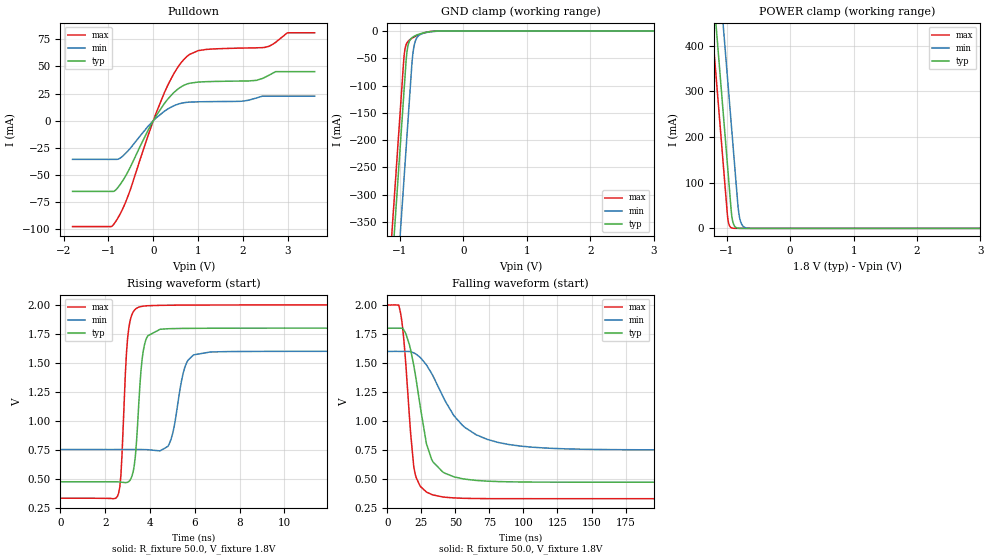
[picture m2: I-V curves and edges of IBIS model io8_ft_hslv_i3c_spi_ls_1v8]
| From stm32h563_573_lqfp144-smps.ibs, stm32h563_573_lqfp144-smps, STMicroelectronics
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[Model]   io8_ft_hslv_i3c_spi_ls_1v8
Model_type I/O_open_drain
Polarity   Non-Inverting
Enable   Active-Low
| CAP_THRESHOLD on pad IOFT is "UDTCAPC" :
| Rising=20.0% of vddiom   Falling=80.0% of vddiom
| C_comp min and max val. don't necessarily correlate with the min and max pvt
| but are the smallest and greatest pad capacitance found.
| var   typ   min   max
C_comp   3.74765pF  3.68522pF  3.87712pF
|C_comp_pulldown   3.74765pF  3.68522pF  3.87712pF
Vinl = 800.0mV
Vinh = 1.0V
Vmeas = 900.0mV   | Reference voltage for timing measurements
Cref  = 50.0pF   | Timing specification test load capacitance value
Rref  = 1.0MOhm   | Timing specification test load resistance value
Vref  = 990.0mV   | Timing specification test load voltage
[Model Spec]
| TIME_THRESHOLD on pin ZII2CV11 is "CMOS" :
| Rising=40.0% of vdd   Falling=60.0% of vdd
Vinl 703.80000mV 631.80000mV 784.80000mV
Vinh 1.06220V 937.20000mV 1.16620V
| variable   typ   min   max
[Temperature Range] 25.0 125.0 -40.0
| variable   typ   min   max
[Voltage Range] 1.8V 1.6V 2.0V
| variable   typ   min   max
[POWER Clamp Reference] 1.8V 1.6V 2.0V
| variable   typ   min   max
[GND Clamp Reference] 0V 0V 0V
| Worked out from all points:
|   slope of the pulldown table from 0 to 0.27 V, typ, clamps not added: 15.8 ohm
|   GND clamp passes 1 mA (typ) near -0.52 V on its own axis
|   POWER clamp passes 1 mA (typ) near -0.84 V on its own axis
|   rising waveform, R_fixture 50.0, V_fixture 1.8V: 20-80 % time 286ps typ, 460ps min, 243ps max; typ from 0.474 V to 1.8 V
|   falling waveform, R_fixture 50.0, V_fixture 1.8V: 20-80 % time 12.1ns typ, 28.6ns min, 6.57ns max; typ from 1.8 V to 0.474 V
[POWER Clamp]
-1.8V     1.518A     1.709A     1.407A
-1.23V    548.8mA    740.2mA    437.5mA
-1.16V    429.8mA    621.2mA    318.5mA
-1.05V    242.8mA    434.2mA    131.5mA
-980mV    123.8mA    315.2mA    17.95mA
-930mV    38.81mA    230.2mA    1.49mA
-910mV    17.82mA    196.2mA    550.8uA
-890mV    8.18mA     162.2mA    203.5uA
-810mV    363.5uA    33.6mA     3.797uA
-770mV    76.62uA    10.47mA    518.8nA
-710mV    7.416uA    1.822mA    26.34nA
3.6V      0A         0A         0A
[GND Clamp]
-1.8V     -1.579A    -1.74A     -1.515A
-1.24V    -627.3mA   -788.3mA   -562.7mA
-1.05V    -304.3mA   -465.3mA   -239.7mA
-940mV    -117.3mA   -278.3mA   -52.69mA
-930mV    -100.3mA   -261.3mA   -40.52mA
-900mV    -50.11mA   -210.3mA   -24.23mA
-880mV    -30.95mA   -176.3mA   -20.02mA
-810mV    -12.18mA   -57.97mA   -13.23mA
-780mV    -9.807mA   -29.1mA    -11.19mA
-690mV    -5.41mA    -7.142mA   -6.184mA
-420mV    -170.4uA   -446.1uA   -81.94uA
3.6V      5.755nA    953.4nA    228.2pA
| variable   typ   min   max
[Pullup Reference] 1.8V 1.6V 2.0V
| variable   typ   min   max
[Pulldown Reference] 0V 0V 0V
[Pulldown]
-1.8V     -65.02mA   -35.56mA   -97.42mA
-940mV    -65.02mA   -35.56mA   -97.42mA
-850mV    -64.17mA   -35.56mA   -93.49mA
-570mV    -47.32mA   -28.01mA   -70.04mA
-120mV    -9.088mA   -5.279mA   -14.07mA
250mV     16.04mA    8.832mA    26.05mA
550mV     29.17mA    15.25mA    49.41mA
780mV     34.17mA    17.07mA    60.14mA
1.18V     35.97mA    17.56mA    65.65mA
2.49V     40mA       22.62mA    67.56mA
2.99V     45.21mA    22.62mA    80.94mA
3.6V      45.21mA    22.62mA    80.94mA
[Ramp]
dV/dt_r 795.76514mV/283.8063ps 508.92555mV/459.40854ps 1.00097V/239.62965ps
dV/dt_f 795.7871mV/11.67148ns 508.95869mV/28.08495ns 1.00099V/6.46824ns
R_load = 50.0
| Removed startup time: 0s 0s 0s  .
| Removed end time: 36.4ns.
[Rising Waveform]
R_fixture   = 50.0
V_fixture   = 1.8V
V_fixture_min = 1.6V
V_fixture_max = 2.0V
0s        473.7mV    751.7mV    331.7mV
2.55ns    473mV      751.8mV    350mV
2.7ns     471mV      751.8mV    525.7mV
3.05ns    474.9mV    751.8mV    1.795V
3.35ns    701.4mV    751.9mV    1.964V
3.6ns     1.437V     751.8mV    1.986V
4.8ns     1.794V     779.2mV    1.997V
5.65ns    1.797V     1.506V     1.999V
6.7ns     1.799V     1.594V     1.999V
36.4ns    1.8V       1.6V       2V
| Removed startup time: 0s 0s 0s  .
| Removed end time: 399.4ns.
[Falling Waveform]
R_fixture   = 50.0
V_fixture   = 1.8V
V_fixture_min = 1.6V
V_fixture_max = 2.0V
0s        1.8V       1.6V       2V
10.1ns    1.8V       1.6V       1.908V
12.85ns   1.77V      1.6V       1.607V
16.3ns    1.655V     1.6V       1.034V
20.35ns   1.419V     1.582V     552.8mV
28.75ns   805.7mV    1.484V     389.3mV
32.6ns    669.3mV    1.41V      367.9mV
55.2ns    503.5mV    964mV      335.3mV
89.65ns   477mV      797.6mV    331.8mV
399.4ns   473.7mV    751.7mV    331.7mV
